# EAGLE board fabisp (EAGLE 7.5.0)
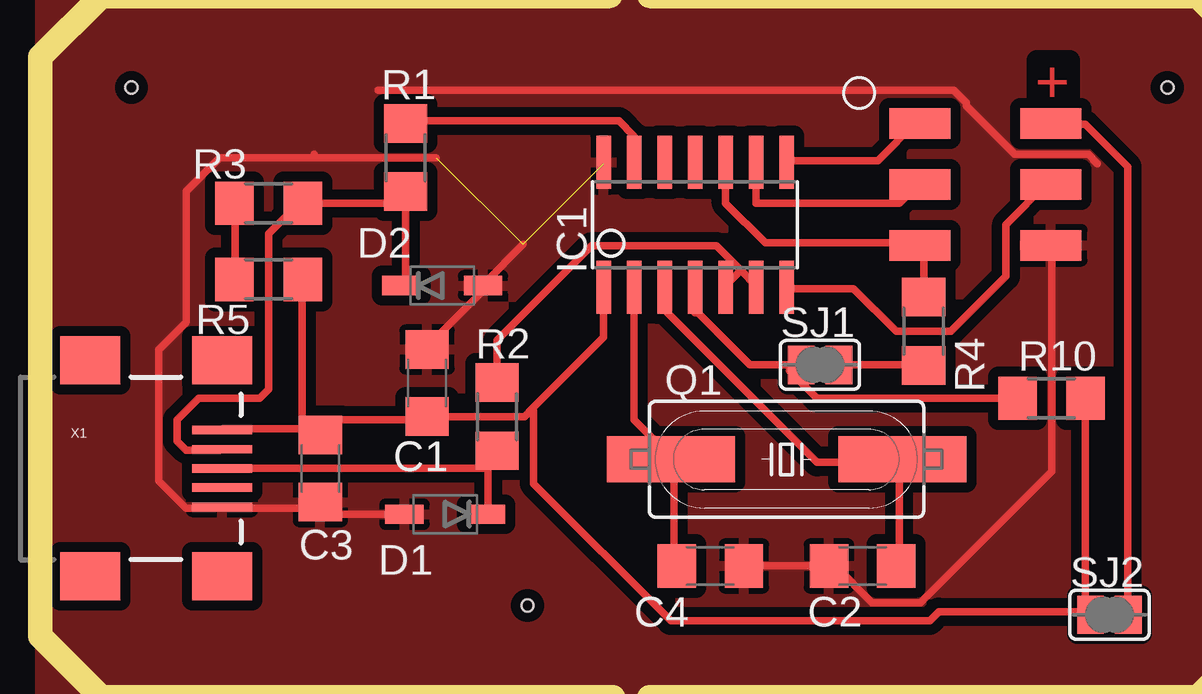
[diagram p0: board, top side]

No outline drawn. Coordinates in mm, seen from the top.
Copper layers (1*16): Top 0.035mm / dielectric 1.5mm / Bottom 0.035mm
Design rules "default *": minimum track width 12mil, minimum drill 24mil, track to track 17mil, track to pad 16mil, pad to pad 16mil, via to via 16mil, smd to smd 0mil, copper to edge 17mil, drill to drill 8mil, minimum pad ring 10mil, minimum via ring 8mil, stop-mask expansion 4mil, vias tented up to drill 0mil, thermal gap 10mil
Holes 0.5 mm at 3.81,24.13 46.99,24.13 20.32,2.54
Milling: 10 lines

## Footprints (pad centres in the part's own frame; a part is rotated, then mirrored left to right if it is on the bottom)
C1206 = smd 1.6 x 1.8: 1 -1.4,0; 2 1.4,0
SOD123 = smd 1.6 x 0.8: ANODE 1.7,0; CATHODE -1.7,0
SOIC14 = smd 0.61 x 2.21: 1 -3.81,-2.603; 2 -2.54,-2.603; 3 -1.27,-2.603; 4 0,-2.603; 5 1.27,-2.603; 6 2.54,-2.603; 7 3.81,-2.603; 8 3.81,2.603; 9 2.54,2.603; 10 1.27,2.603; 11 0,2.603; 12 -1.27,2.603; 13 -2.54,2.603; 14 -3.81,2.603
HC49UP = smd 5.334 x 1.93: 1 -4.826,0; 2 4.826,0
R1206 = smd 1.6 x 1.803: 1 -1.422,0; 2 1.422,0
SJFAB = smd 1.118 x 1.6: 1 -0.787,0; 2 0.787,0
2X3_SMD = smd 2.54 x 1.27: 1 -2.54,2.54; 2 2.92,2.54; 3 -2.54,0; 4 2.92,0; 5 -2.54,-2.54; 6 2.92,-2.54
USB_MINIB = smd 2.5 x 0.35: D+ 3.77,0; D- 3.77,0.8; GND 3.77,-1.6; ID 3.77,-0.8; VBUS 3.77,1.6 | smd 2.5 x 2: GND@1 -1.73,-4.5; GND@2 -1.73,4.5; GND@3 3.77,4.5; GND@4 3.77,-4.5

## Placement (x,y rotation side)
C1  0.1uF  [C1206]  16.13,11.81 90 top
C2  18pF  [C1206]  34.29,4.19 180 top
C3  10uF  [C1206]  11.68,8.26 270 top
C4  18pF  [C1206]  27.94,4.19 0 top
D1  3.3V  [SOD123]  16.89,6.35 180 top
D2  3.3V  [SOD123]  16.76,15.88 0 top
IC1  ATTINY24/44/84-SSU  [SOIC14]  27.3,18.41 0 top
Q1  12MHz  [HC49UP]  31.11,8.64 0 top
R1  49  [R1206]  15.24,21.21 90 top
R2  49  [R1206]  19.05,10.41 90 top
R3  1K  [R1206]  9.53,19.3 180 top
R4  0  [R1206]  36.83,13.97 90 top
R5  499  [R1206]  9.53,16.13 0 top
R10  10K  [R1206]  42.16,11.18 0 top
SJ1  SJFAB  [SJFAB]  32.51,12.57 0 top
SJ2  [SJFAB]  44.58,2.16 0 top
U$1  2X3HEADER  [2X3_SMD]  39.22,20.09 0 top
X1  USB_MINIB  [USB_MINIB]  3.81,8.26 0 top

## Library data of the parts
C1 R1-R3 R10 = rcl-ez
C2-C4 R4 R5 = rcl
D1 D2 = ng
IC1 = attiny24_44_84
Q1 = crystal
SJ1 SJ2 U$1 X1 = mellis

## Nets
D+: IC1.5 IC1.6 R2.2
D-: IC1.13 R1.2
GND: C1.2 C2.2 C3.2 C4.2 D1.ANODE D2.ANODE IC1.14 U$1.6 X1.GND
MISO: IC1.8 U$1.1
MOSI: IC1.7 U$1.4
N$1: D2.CATHODE R1.1 R3.1 X1.D-
N$2: D1.CATHODE R2.1 X1.D+
N$3: R4.1 SJ1.2
N$4: C4.1 IC1.2 Q1.1
N$5: C2.1 IC1.3 Q1.2
N$6: R3.2 R5.1
RESET: IC1.4 R10.1 SJ1.1
RST: IC1.10 R4.2 U$1.5
SCK: IC1.9 U$1.3
VCC: C1.1 C3.1 IC1.1 R5.2 R10.2 SJ2.1 X1.VBUS
VCC': SJ2.2 U$1.2

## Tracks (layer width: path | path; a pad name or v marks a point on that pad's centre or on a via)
D+
  Top 0.305: 29.21,16.51 29.84,15.88 IC1.6 | 29.21,16.51 28.19,17.53 22.99,17.53 19.05,13.59 R2.2 | 29.21,16.51 28.57,15.88 IC1.5
D-
  Top 0.305: 24.77,21.97 IC1.13 24.77,22.1 24.13,22.73 15.24,22.73 R1.2
GND  (2 unrouted)
  Top 0.305: D1.ANODE 12.06,6.35 11.68,6.73 C3.2 11.68,6.6 7.62,6.6 X1.GND 7.49,6.6 6.1,6.6 4.95,7.75 4.95,13.21 6.1,14.35 6.1,19.81 7.49,21.21 11.43,21.21 | C1.2 16.13,13.34 18.41,15.62 18.41,15.88 D2.ANODE 18.54,16 20.13,17.59 | C2.2 C4.2 | C2.2 33.02,4.19 | U$1.6 42.16,17.53 42.16,8.13 36.7,2.67 34.67,2.67 33.15,4.19 C2.2 | 23.5,20.95 IC1.14 | 11.43,21.21 16.51,21.21 | 44.07,20.95 43.69,21.34 40.64,21.34 38.61,23.37 38.61,23.5 38.1,24 14.1,24 | 11.43,21.21 11.43,21.34
  pour Top: 0,27.94 50.8,27.94 50.8,-1.27 0,-1.27
MISO
  Top 0.305: 31.11,21.08 IC1.8 31.24,21.08 34.92,21.08 36.58,22.73 U$1.1
MOSI
  Top 0.305: IC1.7 31.11,15.75 33.91,15.75 35.69,13.97 37.97,13.97 40.26,16.26 40.26,18.41 42.04,20.19 U$1.4
N$1
  Top 0.305: 15.24,16.13 15.11,16 D2.CATHODE 15.24,16.26 R1.1 15.11,19.3 R3.1 10.79,19.3 9.53,18.03 9.53,11.56 9.14,11.18 6.6,11.18 5.71,10.29 5.71,9.4 6.1,9.02 7.49,9.02 X1.D-
N$2
  Top 0.305: D1.CATHODE 18.67,6.35 18.67,8.51 19.05,8.89 R2.1 18.54,8.26 X1.D+
N$3
  Top 0.305: SJ1.2 36.83,12.57 R4.1
N$4
  Top 0.305: C4.1 26.42,4.19 26.42,8.51 Q1.1 26.29,8.76 24.77,10.29 IC1.2
N$5
  Top 0.305: C2.1 35.81,4.19 35.81,8.51 Q1.2 35.69,8.51 32.38,8.51 26.04,14.86 IC1.3
N$6
  Top 0.305: R5.1 8.13,16.13 8.13,19.3 R3.2
RESET
  Top 0.305: IC1.4 27.3,14.86 | IC1.4 27.3,14.73 | SJ1.1 29.59,12.57 27.43,14.73 IC1.4 | SJ1.1 31.24,12.45 | SJ1.1 31.24,12.32 32.38,11.18 R10.1
RST
  Top 0.305: R4.2 36.83,17.4 36.7,17.53 U$1.5 36.58,17.65 30.23,17.65 28.57,19.3 IC1.10
SCK
  Top 0.305: U$1.3 36.58,20.07 35.81,19.3 31.11,19.3 30.61,19.3 29.84,19.3 IC1.9
VCC
  Top 0.305: X1.VBUS 7.62,9.91 11.56,9.91 C3.1 | SJ2.1 43.69,2.16 | 43.56,11.43 R10.2 43.56,11.05 43.56,2.41 SJ2.1 | SJ2.1 43.56,2.29 | C3.1 11.68,9.91 12.06,10.29 16.13,10.29 C1.1 16.26,10.41 20.19,10.41 20.51,10.73 | 20.51,10.73 23.5,13.72 IC1.1 | SJ2.1 43.43,2.29 37.47,2.29 37.08,1.91 26.29,1.91 20.57,7.62 20.57,10.67 20.51,10.73 | R5.2 10.92,16.13 10.92,10.03 C3.1
VCC'
  Top 0.305: U$1.2 42.16,22.61 | U$1.2 42.29,22.61 | SJ2.2 45.34,2.16 45.34,20.83 43.56,22.61 42.42,22.61 U$1.2

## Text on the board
Top: +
